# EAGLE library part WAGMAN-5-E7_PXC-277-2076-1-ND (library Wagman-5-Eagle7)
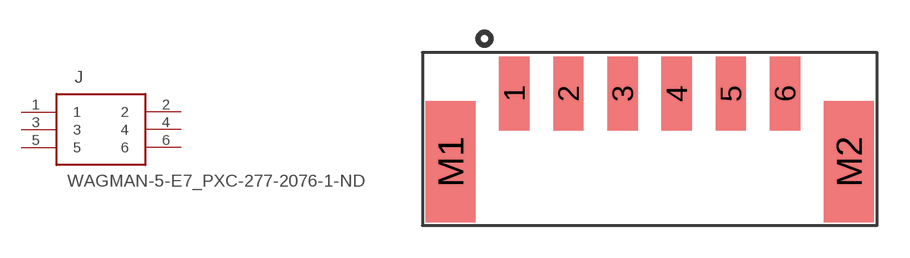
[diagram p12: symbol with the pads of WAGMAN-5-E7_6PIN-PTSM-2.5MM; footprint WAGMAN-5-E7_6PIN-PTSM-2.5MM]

Designator prefix J

## WAGMAN-5-E7_PXC-277-2076-1-ND  [WAGMAN-5-E7_6PIN-PTSM-2.5MM]
1  1
2  2
3  3
4  4
5  5
6  6

## Footprint WAGMAN-5-E7_6PIN-PTSM-2.5MM (pad centres in mm)
smd 1.4 x 3.4: 1 -6.25,0; 2 -3.75,0; 3 -1.25,0; 4 1.25,0; 5 3.75,0; 6 6.25,0
smd 2.3 x 5.6: M1 -9.2,-3.15; M2 9.2,-3.15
